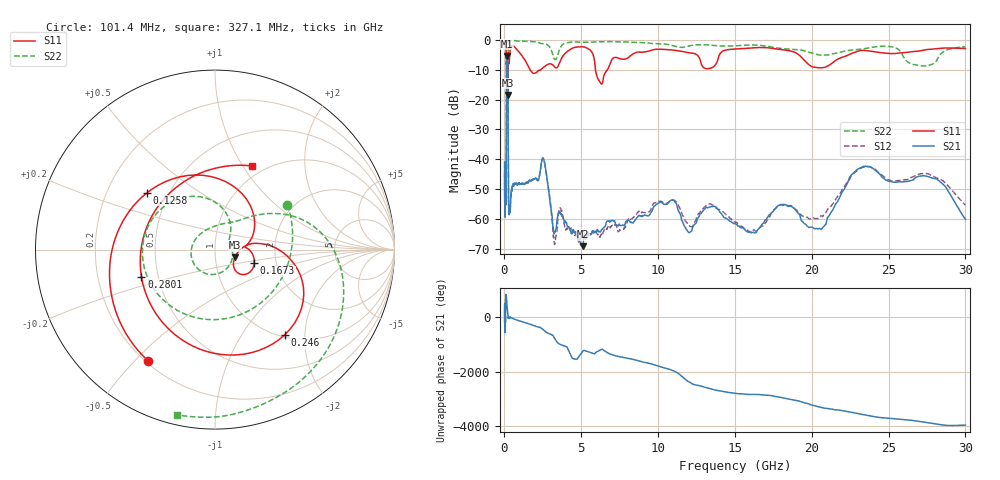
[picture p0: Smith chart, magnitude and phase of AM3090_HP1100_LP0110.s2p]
! Date/Time: Thu, Feb 28, 2019 2:06 PM
! Network Analyzer: Agilent Technologies E8364B Rev: A.07.50.67
! Sweep from 0.010 to 30.000 GHz, 1601 Points, Sweep Type: LOG
! Power Supply: 5.023 V, 0.002 A
# Hz S DB R 50
!freq MagS11 AngS11 MagS21 AngS21 MagS12 AngS12 MagS22 AngS22
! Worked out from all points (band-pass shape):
!   1601 points, 10 MHz to 30 GHz, reference 50 ohm
!   highest |S21| = -5.41 dB at 174.1 MHz (marker M1); lowest = -69.1 dB at 5.103 GHz (marker M2)
!   |S21| within 3 dB of the highest: 141.8 MHz to 215.3 MHz (73.58 MHz wide, 41.2 % of centre)
!   lowest |S11| = -18.5 dB at 201.3 MHz (marker M3), VSWR 1.27, Z = 62.3 - j5.43 ohm
!   |S11| at or under -10 dB: 136.3 MHz to 223.2 MHz (86.86 MHz wide, 48.3 % of centre); 1.669 GHz to 2.36 GHz (691.1 MHz wide, 34.3 % of centre); 5.926 GHz to 6.698 GHz (772.5 MHz wide, 12.2 % of centre)
!   |S22| runs from -21.3 to -0.2 dB; largest |S21 - S12| = 0.011
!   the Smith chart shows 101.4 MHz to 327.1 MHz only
!   S11 on the Smith chart (normalised r, x): 101.4 MHz: 0.21, -0.55; 125.8 MHz: 0.38, +0.32; 167.3 MHz: 1.54, -0.25; 246 MHz: 1.04, -1.58; 280.1 MHz: 0.40, -0.15; 327.1 MHz: 0.87, +1.10
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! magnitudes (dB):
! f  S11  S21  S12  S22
! 10 MHz  -0.2  -40.9  -48.7  -0.6
! 38.04 MHz  -0.4  -56.0  -57.7  -1.3
! 101.4 MHz  -2.8  -53.8  -54.2  -6.5
! 125.8 MHz  -6.1  -24.8  -24.7  -7.8
! 144.7 MHz  -14.7  -7.4  -7.4  -18.6
! 167.3 MHz  -12.7  -5.5  -5.4  -18.1
! 174.1 MHz  -12.6  -5.4  -5.4  -17.0
! 201.3 MHz  -18.5  -6.3  -6.3  -18.4
! 224.8 MHz  -9.4  -12.6  -12.5  -11.1
! 246 MHz  -4.2  -37.8  -37.1  -2.8
! 280.1 MHz  -7.2  -57.1  -55.8  -1.0
! 327.1 MHz  -5.9  -57.0  -57.2  -0.5
! 550.5 MHz  -2.0  -49.2  -48.9  -0.3
! 2.084 GHz  -10.9  -46.5  -46.7  -0.7
! 2.545 GHz  -9.1  -39.9  -40.0  -1.3
! 3.253 GHz  -9.0  -64.6  -68.6  -6.4
! 5.103 GHz  -2.3  -69.1  -66.4  -0.8
! 6.202 GHz  -14.0  -64.3  -66.2  -0.6
! 7.926 GHz  -6.3  -60.7  -62.3  -0.7
! 20.2 GHz  -9.2  -63.3  -60.0  -4.7
! 23.48 GHz  -3.5  -42.3  -42.5  -2.9
! 30 GHz  -2.9  -60.1  -55.4  -2.3
